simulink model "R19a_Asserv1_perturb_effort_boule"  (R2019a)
settings: Solver=ode15s  StartTime=0.0  StopTime=1  RelTol=1e-3  EnableMultiTasking=on
undefined symbols (not defined in the file): deg, kg, m, manette1_Défaut_sldprt, manette2_Défaut_sldprt, mm, N, rad, s, sigbuilder_block, STL, X, Y, Z
libraries: sm_lib x460, fl_lib x45, nesl_utility x23, simulink x3
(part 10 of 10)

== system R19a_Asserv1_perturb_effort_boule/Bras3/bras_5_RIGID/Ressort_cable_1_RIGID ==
  ReferenceFrame : sm_lib/Frames and Transforms/Reference Frame
  Solid : sm_lib/Body Elements/Solid  InertiaType=Custom  Mass=0.0011765814520035881  MassUnits=kg  CenterOfMass=[0.086849073647483815 -0.00090479521327996976 6.9508776157243597]  CenterOfMassUnits=mm  MomentsOfInertia=[0.034952381374405594 0.034338972761516762 0.0097063586011258158]  MomentsOfInertiaUnits=kg*mm^2  ProductsOfInertia=[0.00037229322226744533 1.6947615167207185e-06 2.0937803976811866e-06]  ProductsOfInertiaUnits=kg*mm^2  BasedOnType=Density  Density=1000  DensityUnits=kg/(m^3)  DoExposeReferenceFrame=on  SerializedFrames=<Frames/>  GraphicType=FromGeometry  MarkerShape=Sphere  MarkerSize=10  MarkerSizeUnits=m  GraphicVisPropType=SimpleVisualProperties  GraphicDiffuseColor=[0.6470588235294118 0.61960784313725492 0.58823529411764708]  GraphicSpecularColor=[0.5 0.5 0.5 1.0]  GraphicAmbientColor=[0.15 0.15 0.15 1.0]  GraphicEmissiveColor=[0.0 0.0 0.0 1.0]  GraphicShininess=75  GraphicOpacity=1  GeometryShape=FromFile  RectangleSize=[1 1]  RectangleSizeUnits=m  BrickDimensions=[1 1 1]  BrickDimensionUnits=m  CylinderRadius=1  CylinderRadiusUnits=m  CylinderLength=1  CylinderLengthUnits=m  SphereRadius=1  SphereRadiusUnits=m  EllipsoidRadii=[1 1 1]  EllipsoidRadiiUnits=m  ExtrusionCrossSection=[1 1; -1 1; -1 -1; 1 -1]  ExtrusionCrossSectionUnits=m  ExtrusionLength=1  ExtrusionLengthUnits=m  PolygonNumSides=3  PolygonOuterRadius=1  PolygonOuterRadiusUnits=m  ExtGeomFileType=STL  ExtGeomFileName=\STL\Ressort cable_Défaut_sldprt.STL  ExtGeomFileUnits=mm  RevolutionCrossSection=[1 1; 1 -1; 2 -1; 2 1]  RevolutionCrossSectionUnits=m  RevolutionExtent=Full  RevolutionAngle=180  RevolutionAngleUnits=deg
  F : PMIOPort  Side=Left
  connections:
  Solid/RConn1 -- ReferenceFrame/RConn1 -- F/RConn1

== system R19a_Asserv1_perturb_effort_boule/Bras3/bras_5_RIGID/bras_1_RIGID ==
  ReferenceFrame : sm_lib/Frames and Transforms/Reference Frame
  Solid : sm_lib/Body Elements/Solid  InertiaType=Custom  Mass=0.06566875822643542  MassUnits=kg  CenterOfMass=[23.925748169887701 -4.7774352723885904 0.0071346362933715022]  CenterOfMassUnits=mm  MomentsOfInertia=[75.153076467382206 23.577652078949701 94.231108050856861]  MomentsOfInertiaUnits=kg*mm^2  ProductsOfInertia=[0.01532312637695204 0.0017211125494294708 -5.8798668472039237]  ProductsOfInertiaUnits=kg*mm^2  BasedOnType=Density  Density=1000  DensityUnits=kg/(m^3)  DoExposeReferenceFrame=on  SerializedFrames=<Frames/>  GraphicType=FromGeometry  MarkerShape=Sphere  MarkerSize=10  MarkerSizeUnits=m  GraphicVisPropType=SimpleVisualProperties  GraphicDiffuseColor=[1.0 1.0 0.0]  GraphicSpecularColor=[0.5 0.5 0.5 1.0]  GraphicAmbientColor=[0.15 0.15 0.15 1.0]  GraphicEmissiveColor=[0.0 0.0 0.0 1.0]  GraphicShininess=75  GraphicOpacity=1  GeometryShape=FromFile  RectangleSize=[1 1]  RectangleSizeUnits=m  BrickDimensions=[1 1 1]  BrickDimensionUnits=m  CylinderRadius=1  CylinderRadiusUnits=m  CylinderLength=1  CylinderLengthUnits=m  SphereRadius=1  SphereRadiusUnits=m  EllipsoidRadii=[1 1 1]  EllipsoidRadiiUnits=m  ExtrusionCrossSection=[1 1; -1 1; -1 -1; 1 -1]  ExtrusionCrossSectionUnits=m  ExtrusionLength=1  ExtrusionLengthUnits=m  PolygonNumSides=3  PolygonOuterRadius=1  PolygonOuterRadiusUnits=m  ExtGeomFileType=STL  ExtGeomFileName=\STL\bras_Défaut_sldprt.STL  ExtGeomFileUnits=mm  RevolutionCrossSection=[1 1; 1 -1; 2 -1; 2 1]  RevolutionCrossSectionUnits=m  RevolutionExtent=Full  RevolutionAngle=180  RevolutionAngleUnits=deg
  F : PMIOPort  Side=Left
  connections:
  Solid/RConn1 -- ReferenceFrame/RConn1 -- F/RConn1

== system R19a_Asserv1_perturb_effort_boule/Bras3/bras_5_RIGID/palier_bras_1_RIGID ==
  ReferenceFrame : sm_lib/Frames and Transforms/Reference Frame
  Solid : sm_lib/Body Elements/Solid  InertiaType=Custom  Mass=0.00017920168094851793  MassUnits=kg  CenterOfMass=[-178.32667601154176 39.825618202078154 -20.980989744703667]  CenterOfMassUnits=mm  MomentsOfInertia=[0.0018602253674838991 0.0012789874237151958 0.0012789874237151961]  MomentsOfInertiaUnits=kg*mm^2  ProductsOfInertia=[0 0 0]  ProductsOfInertiaUnits=kg*mm^2  BasedOnType=Density  Density=1000  DensityUnits=kg/(m^3)  DoExposeReferenceFrame=on  SerializedFrames=<Frames/>  GraphicType=FromGeometry  MarkerShape=Sphere  MarkerSize=10  MarkerSizeUnits=m  GraphicVisPropType=SimpleVisualProperties  GraphicDiffuseColor=[1 1 1]  GraphicSpecularColor=[0.5 0.5 0.5 1.0]  GraphicAmbientColor=[0.15 0.15 0.15 1.0]  GraphicEmissiveColor=[0.0 0.0 0.0 1.0]  GraphicShininess=75  GraphicOpacity=1  GeometryShape=FromFile  RectangleSize=[1 1]  RectangleSizeUnits=m  BrickDimensions=[1 1 1]  BrickDimensionUnits=m  CylinderRadius=1  CylinderRadiusUnits=m  CylinderLength=1  CylinderLengthUnits=m  SphereRadius=1  SphereRadiusUnits=m  EllipsoidRadii=[1 1 1]  EllipsoidRadiiUnits=m  ExtrusionCrossSection=[1 1; -1 1; -1 -1; 1 -1]  ExtrusionCrossSectionUnits=m  ExtrusionLength=1  ExtrusionLengthUnits=m  PolygonNumSides=3  PolygonOuterRadius=1  PolygonOuterRadiusUnits=m  ExtGeomFileType=STL  ExtGeomFileName=\STL\palier bras_Défaut_sldprt.STL  ExtGeomFileUnits=mm  RevolutionCrossSection=[1 1; 1 -1; 2 -1; 2 1]  RevolutionCrossSectionUnits=m  RevolutionExtent=Full  RevolutionAngle=180  RevolutionAngleUnits=deg
  F : PMIOPort  Side=Left
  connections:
  Solid/RConn1 -- ReferenceFrame/RConn1 -- F/RConn1

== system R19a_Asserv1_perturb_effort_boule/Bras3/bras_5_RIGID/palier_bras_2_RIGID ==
  ReferenceFrame : sm_lib/Frames and Transforms/Reference Frame
  Solid : sm_lib/Body Elements/Solid  InertiaType=Custom  Mass=0.00017920168094851793  MassUnits=kg  CenterOfMass=[-178.32667601154176 39.825618202078154 -20.980989744703667]  CenterOfMassUnits=mm  MomentsOfInertia=[0.0018602253674838991 0.0012789874237151958 0.0012789874237151961]  MomentsOfInertiaUnits=kg*mm^2  ProductsOfInertia=[0 0 0]  ProductsOfInertiaUnits=kg*mm^2  BasedOnType=Density  Density=1000  DensityUnits=kg/(m^3)  DoExposeReferenceFrame=on  SerializedFrames=<Frames/>  GraphicType=FromGeometry  MarkerShape=Sphere  MarkerSize=10  MarkerSizeUnits=m  GraphicVisPropType=SimpleVisualProperties  GraphicDiffuseColor=[1 1 1]  GraphicSpecularColor=[0.5 0.5 0.5 1.0]  GraphicAmbientColor=[0.15 0.15 0.15 1.0]  GraphicEmissiveColor=[0.0 0.0 0.0 1.0]  GraphicShininess=75  GraphicOpacity=1  GeometryShape=FromFile  RectangleSize=[1 1]  RectangleSizeUnits=m  BrickDimensions=[1 1 1]  BrickDimensionUnits=m  CylinderRadius=1  CylinderRadiusUnits=m  CylinderLength=1  CylinderLengthUnits=m  SphereRadius=1  SphereRadiusUnits=m  EllipsoidRadii=[1 1 1]  EllipsoidRadiiUnits=m  ExtrusionCrossSection=[1 1; -1 1; -1 -1; 1 -1]  ExtrusionCrossSectionUnits=m  ExtrusionLength=1  ExtrusionLengthUnits=m  PolygonNumSides=3  PolygonOuterRadius=1  PolygonOuterRadiusUnits=m  ExtGeomFileType=STL  ExtGeomFileName=\STL\palier bras_Défaut_sldprt.STL  ExtGeomFileUnits=mm  RevolutionCrossSection=[1 1; 1 -1; 2 -1; 2 1]  RevolutionCrossSectionUnits=m  RevolutionExtent=Full  RevolutionAngle=180  RevolutionAngleUnits=deg
  F : PMIOPort  Side=Left
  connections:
  Solid/RConn1 -- ReferenceFrame/RConn1 -- F/RConn1

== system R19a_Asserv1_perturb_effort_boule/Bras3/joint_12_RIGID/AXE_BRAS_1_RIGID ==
  ReferenceFrame : sm_lib/Frames and Transforms/Reference Frame
  Solid : sm_lib/Body Elements/Solid  InertiaType=Custom  Mass=0.0015327306958088996  MassUnits=kg  CenterOfMass=[0 0 0]  CenterOfMassUnits=mm  MomentsOfInertia=[0.11359646260705632 0.11359646260705632 0.0017137152305883286]  MomentsOfInertiaUnits=kg*mm^2  ProductsOfInertia=[0 0 0]  ProductsOfInertiaUnits=kg*mm^2  BasedOnType=Density  Density=1000  DensityUnits=kg/(m^3)  DoExposeReferenceFrame=on  SerializedFrames=<Frames/>  GraphicType=FromGeometry  MarkerShape=Sphere  MarkerSize=10  MarkerSizeUnits=m  GraphicVisPropType=SimpleVisualProperties  GraphicDiffuseColor=[0.6470588235294118 0.61960784313725492 0.58823529411764708]  GraphicSpecularColor=[0.5 0.5 0.5 1.0]  GraphicAmbientColor=[0.15 0.15 0.15 1.0]  GraphicEmissiveColor=[0.0 0.0 0.0 1.0]  GraphicShininess=75  GraphicOpacity=1  GeometryShape=FromFile  RectangleSize=[1 1]  RectangleSizeUnits=m  BrickDimensions=[1 1 1]  BrickDimensionUnits=m  CylinderRadius=1  CylinderRadiusUnits=m  CylinderLength=1  CylinderLengthUnits=m  SphereRadius=1  SphereRadiusUnits=m  EllipsoidRadii=[1 1 1]  EllipsoidRadiiUnits=m  ExtrusionCrossSection=[1 1; -1 1; -1 -1; 1 -1]  ExtrusionCrossSectionUnits=m  ExtrusionLength=1  ExtrusionLengthUnits=m  PolygonNumSides=3  PolygonOuterRadius=1  PolygonOuterRadiusUnits=m  ExtGeomFileType=STL  ExtGeomFileName=\STL\AXE BRAS_Défaut_sldprt.STL  ExtGeomFileUnits=mm  RevolutionCrossSection=[1 1; 1 -1; 2 -1; 2 1]  RevolutionCrossSectionUnits=m  RevolutionExtent=Full  RevolutionAngle=180  RevolutionAngleUnits=deg
  F : PMIOPort  Side=Left
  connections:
  Solid/RConn1 -- ReferenceFrame/RConn1 -- F/RConn1

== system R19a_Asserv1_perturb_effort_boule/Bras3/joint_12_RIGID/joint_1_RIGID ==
  ReferenceFrame : sm_lib/Frames and Transforms/Reference Frame
  Solid : sm_lib/Body Elements/Solid  InertiaType=Custom  Mass=0.0062454336323428689  MassUnits=kg  CenterOfMass=[-4.7519597301086606e-06 14.873568128586268 0.2827021501004604]  CenterOfMassUnits=mm  MomentsOfInertia=[0.43544209184236687 0.81590742360241675 0.91424830357082487]  MomentsOfInertiaUnits=kg*mm^2  ProductsOfInertia=[0.0068320776316595647 -4.173068650825101e-06 -7.5142319098046527e-07]  ProductsOfInertiaUnits=kg*mm^2  BasedOnType=Density  Density=1000  DensityUnits=kg/(m^3)  DoExposeReferenceFrame=on  SerializedFrames=<Frames/>  GraphicType=FromGeometry  MarkerShape=Sphere  MarkerSize=10  MarkerSizeUnits=m  GraphicVisPropType=SimpleVisualProperties  GraphicDiffuseColor=[1 1 1]  GraphicSpecularColor=[0.5 0.5 0.5 1.0]  GraphicAmbientColor=[0.15 0.15 0.15 1.0]  GraphicEmissiveColor=[0.0 0.0 0.0 1.0]  GraphicShininess=75  GraphicOpacity=1  GeometryShape=FromFile  RectangleSize=[1 1]  RectangleSizeUnits=m  BrickDimensions=[1 1 1]  BrickDimensionUnits=m  CylinderRadius=1  CylinderRadiusUnits=m  CylinderLength=1  CylinderLengthUnits=m  SphereRadius=1  SphereRadiusUnits=m  EllipsoidRadii=[1 1 1]  EllipsoidRadiiUnits=m  ExtrusionCrossSection=[1 1; -1 1; -1 -1; 1 -1]  ExtrusionCrossSectionUnits=m  ExtrusionLength=1  ExtrusionLengthUnits=m  PolygonNumSides=3  PolygonOuterRadius=1  PolygonOuterRadiusUnits=m  ExtGeomFileType=STL  ExtGeomFileName=\STL\joint_Défaut_sldprt.STL  ExtGeomFileUnits=mm  RevolutionCrossSection=[1 1; 1 -1; 2 -1; 2 1]  RevolutionCrossSectionUnits=m  RevolutionExtent=Full  RevolutionAngle=180  RevolutionAngleUnits=deg
  F : PMIOPort  Side=Left
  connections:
  Solid/RConn1 -- ReferenceFrame/RConn1 -- F/RConn1

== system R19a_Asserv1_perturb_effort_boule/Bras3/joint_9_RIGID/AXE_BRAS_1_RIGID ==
  ReferenceFrame : sm_lib/Frames and Transforms/Reference Frame
  Solid : sm_lib/Body Elements/Solid  InertiaType=Custom  Mass=0.0015327306958088996  MassUnits=kg  CenterOfMass=[0 0 0]  CenterOfMassUnits=mm  MomentsOfInertia=[0.11359646260705632 0.11359646260705632 0.0017137152305883286]  MomentsOfInertiaUnits=kg*mm^2  ProductsOfInertia=[0 0 0]  ProductsOfInertiaUnits=kg*mm^2  BasedOnType=Density  Density=1000  DensityUnits=kg/(m^3)  DoExposeReferenceFrame=on  SerializedFrames=<Frames/>  GraphicType=FromGeometry  MarkerShape=Sphere  MarkerSize=10  MarkerSizeUnits=m  GraphicVisPropType=SimpleVisualProperties  GraphicDiffuseColor=[0.6470588235294118 0.61960784313725492 0.58823529411764708]  GraphicSpecularColor=[0.5 0.5 0.5 1.0]  GraphicAmbientColor=[0.15 0.15 0.15 1.0]  GraphicEmissiveColor=[0.0 0.0 0.0 1.0]  GraphicShininess=75  GraphicOpacity=1  GeometryShape=FromFile  RectangleSize=[1 1]  RectangleSizeUnits=m  BrickDimensions=[1 1 1]  BrickDimensionUnits=m  CylinderRadius=1  CylinderRadiusUnits=m  CylinderLength=1  CylinderLengthUnits=m  SphereRadius=1  SphereRadiusUnits=m  EllipsoidRadii=[1 1 1]  EllipsoidRadiiUnits=m  ExtrusionCrossSection=[1 1; -1 1; -1 -1; 1 -1]  ExtrusionCrossSectionUnits=m  ExtrusionLength=1  ExtrusionLengthUnits=m  PolygonNumSides=3  PolygonOuterRadius=1  PolygonOuterRadiusUnits=m  ExtGeomFileType=STL  ExtGeomFileName=\STL\AXE BRAS_Défaut_sldprt.STL  ExtGeomFileUnits=mm  RevolutionCrossSection=[1 1; 1 -1; 2 -1; 2 1]  RevolutionCrossSectionUnits=m  RevolutionExtent=Full  RevolutionAngle=180  RevolutionAngleUnits=deg
  F : PMIOPort  Side=Left
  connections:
  Solid/RConn1 -- ReferenceFrame/RConn1 -- F/RConn1

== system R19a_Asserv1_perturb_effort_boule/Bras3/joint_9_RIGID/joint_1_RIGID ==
  ReferenceFrame : sm_lib/Frames and Transforms/Reference Frame
  Solid : sm_lib/Body Elements/Solid  InertiaType=Custom  Mass=0.0062454336323428689  MassUnits=kg  CenterOfMass=[-4.7519597301086606e-06 14.873568128586268 0.2827021501004604]  CenterOfMassUnits=mm  MomentsOfInertia=[0.43544209184236687 0.81590742360241675 0.91424830357082487]  MomentsOfInertiaUnits=kg*mm^2  ProductsOfInertia=[0.0068320776316595647 -4.173068650825101e-06 -7.5142319098046527e-07]  ProductsOfInertiaUnits=kg*mm^2  BasedOnType=Density  Density=1000  DensityUnits=kg/(m^3)  DoExposeReferenceFrame=on  SerializedFrames=<Frames/>  GraphicType=FromGeometry  MarkerShape=Sphere  MarkerSize=10  MarkerSizeUnits=m  GraphicVisPropType=SimpleVisualProperties  GraphicDiffuseColor=[1 1 1]  GraphicSpecularColor=[0.5 0.5 0.5 1.0]  GraphicAmbientColor=[0.15 0.15 0.15 1.0]  GraphicEmissiveColor=[0.0 0.0 0.0 1.0]  GraphicShininess=75  GraphicOpacity=1  GeometryShape=FromFile  RectangleSize=[1 1]  RectangleSizeUnits=m  BrickDimensions=[1 1 1]  BrickDimensionUnits=m  CylinderRadius=1  CylinderRadiusUnits=m  CylinderLength=1  CylinderLengthUnits=m  SphereRadius=1  SphereRadiusUnits=m  EllipsoidRadii=[1 1 1]  EllipsoidRadiiUnits=m  ExtrusionCrossSection=[1 1; -1 1; -1 -1; 1 -1]  ExtrusionCrossSectionUnits=m  ExtrusionLength=1  ExtrusionLengthUnits=m  PolygonNumSides=3  PolygonOuterRadius=1  PolygonOuterRadiusUnits=m  ExtGeomFileType=STL  ExtGeomFileName=\STL\joint_Défaut_sldprt.STL  ExtGeomFileUnits=mm  RevolutionCrossSection=[1 1; 1 -1; 2 -1; 2 1]  RevolutionCrossSectionUnits=m  RevolutionExtent=Full  RevolutionAngle=180  RevolutionAngleUnits=deg
  F : PMIOPort  Side=Left
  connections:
  Solid/RConn1 -- ReferenceFrame/RConn1 -- F/RConn1

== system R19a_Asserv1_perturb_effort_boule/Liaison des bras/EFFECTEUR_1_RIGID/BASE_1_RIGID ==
  ReferenceFrame : sm_lib/Frames and Transforms/Reference Frame
  Solid : sm_lib/Body Elements/Solid  InertiaType=Custom  Mass=0.028238598075005058  MassUnits=kg  CenterOfMass=[-0.50940754911928388 -1.6318221689243708 -4.5607511741024656]  CenterOfMassUnits=mm  MomentsOfInertia=[8.5842414198569479 7.5819347196129669 14.129620619032369]  MomentsOfInertiaUnits=kg*mm^2  ProductsOfInertia=[-0.29549774773685261 -0.082418003511546406 -0.14811223553088118]  ProductsOfInertiaUnits=kg*mm^2  BasedOnType=Density  Density=1000  DensityUnits=kg/(m^3)  DoExposeReferenceFrame=on  SerializedFrames=<Frames/>  GraphicType=FromGeometry  MarkerShape=Sphere  MarkerSize=10  MarkerSizeUnits=m  GraphicVisPropType=SimpleVisualProperties  GraphicDiffuseColor=[1.0 1.0 1.0]  GraphicSpecularColor=[0.5 0.5 0.5 1.0]  GraphicAmbientColor=[0.15 0.15 0.15 1.0]  GraphicEmissiveColor=[0.0 0.0 0.0 1.0]  GraphicShininess=75  GraphicOpacity=1  GeometryShape=FromFile  RectangleSize=[1 1]  RectangleSizeUnits=m  BrickDimensions=[1 1 1]  BrickDimensionUnits=m  CylinderRadius=1  CylinderRadiusUnits=m  CylinderLength=1  CylinderLengthUnits=m  SphereRadius=1  SphereRadiusUnits=m  EllipsoidRadii=[1 1 1]  EllipsoidRadiiUnits=m  ExtrusionCrossSection=[1 1; -1 1; -1 -1; 1 -1]  ExtrusionCrossSectionUnits=m  ExtrusionLength=1  ExtrusionLengthUnits=m  PolygonNumSides=3  PolygonOuterRadius=1  PolygonOuterRadiusUnits=m  ExtGeomFileType=STL  ExtGeomFileName=\STL\BASE_Défaut_sldprt.STL  ExtGeomFileUnits=mm  RevolutionCrossSection=[1 1; 1 -1; 2 -1; 2 1]  RevolutionCrossSectionUnits=m  RevolutionExtent=Full  RevolutionAngle=180  RevolutionAngleUnits=deg
  F : PMIOPort  Side=Left
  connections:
  Solid/RConn1 -- ReferenceFrame/RConn1 -- F/RConn1

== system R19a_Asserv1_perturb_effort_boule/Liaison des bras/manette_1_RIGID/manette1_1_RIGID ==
  ReferenceFrame : sm_lib/Frames and Transforms/Reference Frame
  Solid : sm_lib/Body Elements/Solid  InertiaType=Custom  Mass=0.021495200046783486  MassUnits=kg  CenterOfMass=[-1.4897475291331288 1.1324325333899619 3.6124835128376875]  CenterOfMassUnits=mm  MomentsOfInertia=[5.4184345928892519 5.4614392106741905 10.048915162120133]  MomentsOfInertiaUnits=kg*mm^2  ProductsOfInertia=[-0.010452851512005331 -0.0018797921399214363 0.024517118393881449]  ProductsOfInertiaUnits=kg*mm^2  BasedOnType=Density  Density=1000  DensityUnits=kg/(m^3)  DoExposeReferenceFrame=on  SerializedFrames=<Frames/>  GraphicType=FromGeometry  MarkerShape=Sphere  MarkerSize=10  MarkerSizeUnits=m  GraphicVisPropType=SimpleVisualProperties  GraphicDiffuseColor=[0.8 0.8 0.8]  GraphicSpecularColor=[0.5 0.5 0.5 1.0]  GraphicAmbientColor=[0.15 0.15 0.15 1.0]  GraphicEmissiveColor=[0.0 0.0 0.0 1.0]  GraphicShininess=75  GraphicOpacity=1  GeometryShape=FromFile  RectangleSize=[1 1]  RectangleSizeUnits=m  BrickDimensions=[1 1 1]  BrickDimensionUnits=m  CylinderRadius=1  CylinderRadiusUnits=m  CylinderLength=1  CylinderLengthUnits=m  SphereRadius=1  SphereRadiusUnits=m  EllipsoidRadii=[1 1 1]  EllipsoidRadiiUnits=m  ExtrusionCrossSection=[1 1; -1 1; -1 -1; 1 -1]  ExtrusionCrossSectionUnits=m  ExtrusionLength=1  ExtrusionLengthUnits=m  PolygonNumSides=3  PolygonOuterRadius=1  PolygonOuterRadiusUnits=m  ExtGeomFileType=STL  ExtGeomFileName=\STL\manette1_Défaut_sldprt.STL  ExtGeomFileUnits=mm  RevolutionCrossSection=[1 1; 1 -1; 2 -1; 2 1]  RevolutionCrossSectionUnits=m  RevolutionExtent=Full  RevolutionAngle=180  RevolutionAngleUnits=deg
  F : PMIOPort  Side=Left
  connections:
  Solid/RConn1 -- ReferenceFrame/RConn1 -- F/RConn1

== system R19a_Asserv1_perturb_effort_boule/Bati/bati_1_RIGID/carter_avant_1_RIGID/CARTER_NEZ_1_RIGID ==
  ReferenceFrame : sm_lib/Frames and Transforms/Reference Frame
  Solid : sm_lib/Body Elements/Solid  InertiaType=Custom  Mass=0.023684568109850399  MassUnits=kg  CenterOfMass=[17.102684932647009 114.0476537917955 1.3404873933864438]  CenterOfMassUnits=mm  MomentsOfInertia=[16.43130676036915 32.571595129912247 16.431105891514132]  MomentsOfInertiaUnits=kg*mm^2  ProductsOfInertia=[-3.788014627850142e-05 -4.8452777139477129e-05 -5.4026210558728518e-06]  ProductsOfInertiaUnits=kg*mm^2  BasedOnType=Density  Density=1000  DensityUnits=kg/(m^3)  DoExposeReferenceFrame=on  SerializedFrames=<Frames/>  GraphicType=FromGeometry  MarkerShape=Sphere  MarkerSize=10  MarkerSizeUnits=m  GraphicVisPropType=SimpleVisualProperties  GraphicDiffuseColor=[0.75294117647058822 0.75294117647058822 0.75294117647058822]  GraphicSpecularColor=[0.5 0.5 0.5 1.0]  GraphicAmbientColor=[0.15 0.15 0.15 1.0]  GraphicEmissiveColor=[0.0 0.0 0.0 1.0]  GraphicShininess=75  GraphicOpacity=1  GeometryShape=FromFile  RectangleSize=[1 1]  RectangleSizeUnits=m  BrickDimensions=[1 1 1]  BrickDimensionUnits=m  CylinderRadius=1  CylinderRadiusUnits=m  CylinderLength=1  CylinderLengthUnits=m  SphereRadius=1  SphereRadiusUnits=m  EllipsoidRadii=[1 1 1]  EllipsoidRadiiUnits=m  ExtrusionCrossSection=[1 1; -1 1; -1 -1; 1 -1]  ExtrusionCrossSectionUnits=m  ExtrusionLength=1  ExtrusionLengthUnits=m  PolygonNumSides=3  PolygonOuterRadius=1  PolygonOuterRadiusUnits=m  ExtGeomFileType=STL  ExtGeomFileName=\STL\CARTER NEZ_Défaut_sldprt.STL  ExtGeomFileUnits=mm  RevolutionCrossSection=[1 1; 1 -1; 2 -1; 2 1]  RevolutionCrossSectionUnits=m  RevolutionExtent=Full  RevolutionAngle=180  RevolutionAngleUnits=deg
  F : PMIOPort  Side=Left
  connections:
  Solid/RConn1 -- ReferenceFrame/RConn1 -- F/RConn1

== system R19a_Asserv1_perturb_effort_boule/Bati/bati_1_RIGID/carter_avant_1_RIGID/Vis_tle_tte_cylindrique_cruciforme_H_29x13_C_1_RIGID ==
  ReferenceFrame : sm_lib/Frames and Transforms/Reference Frame
  Solid : sm_lib/Body Elements/Solid  InertiaType=Custom  Mass=8.3821869835456372e-05  MassUnits=kg  CenterOfMass=[4.9478681581074904 0.00064910481891303923 -0.0013634218224953438]  CenterOfMassUnits=mm  MomentsOfInertia=[0.00016543197172893975 0.0014334630955093895 0.0014333390308476422]  MomentsOfInertiaUnits=kg*mm^2  ProductsOfInertia=[-5.4062904633677868e-09 -1.3111174919527308e-07 6.0713893531177014e-07]  ProductsOfInertiaUnits=kg*mm^2  BasedOnType=Density  Density=1000  DensityUnits=kg/(m^3)  DoExposeReferenceFrame=on  SerializedFrames=<Frames/>  GraphicType=FromGeometry  MarkerShape=Sphere  MarkerSize=10  MarkerSizeUnits=m  GraphicVisPropType=SimpleVisualProperties  GraphicDiffuseColor=[0.75294117647058822 0.75294117647058822 0.75294117647058822]  GraphicSpecularColor=[0.5 0.5 0.5 1.0]  GraphicAmbientColor=[0.15 0.15 0.15 1.0]  GraphicEmissiveColor=[0.0 0.0 0.0 1.0]  GraphicShininess=75  GraphicOpacity=1  GeometryShape=FromFile  RectangleSize=[1 1]  RectangleSizeUnits=m  BrickDimensions=[1 1 1]  BrickDimensionUnits=m  CylinderRadius=1  CylinderRadiusUnits=m  CylinderLength=1  CylinderLengthUnits=m  SphereRadius=1  SphereRadiusUnits=m  EllipsoidRadii=[1 1 1]  EllipsoidRadiiUnits=m  ExtrusionCrossSection=[1 1; -1 1; -1 -1; 1 -1]  ExtrusionCrossSectionUnits=m  ExtrusionLength=1  ExtrusionLengthUnits=m  PolygonNumSides=3  PolygonOuterRadius=1  PolygonOuterRadiusUnits=m  ExtGeomFileType=STL  ExtGeomFileName=\STL\Vis à tôle tête cylindrique cruciforme H 2-9x13 - C_Réaliste_sldprt.STL  ExtGeomFileUnits=mm  RevolutionCrossSection=[1 1; 1 -1; 2 -1; 2 1]  RevolutionCrossSectionUnits=m  RevolutionExtent=Full  RevolutionAngle=180  RevolutionAngleUnits=deg
  F : PMIOPort  Side=Left
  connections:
  Solid/RConn1 -- ReferenceFrame/RConn1 -- F/RConn1

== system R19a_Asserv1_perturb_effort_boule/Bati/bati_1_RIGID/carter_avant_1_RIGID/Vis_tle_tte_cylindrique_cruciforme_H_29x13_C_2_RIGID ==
  ReferenceFrame : sm_lib/Frames and Transforms/Reference Frame
  Solid : sm_lib/Body Elements/Solid  InertiaType=Custom  Mass=8.3821869835456372e-05  MassUnits=kg  CenterOfMass=[4.9478681581074904 0.00064910481891303923 -0.0013634218224953438]  CenterOfMassUnits=mm  MomentsOfInertia=[0.00016543197172893975 0.0014334630955093895 0.0014333390308476422]  MomentsOfInertiaUnits=kg*mm^2  ProductsOfInertia=[-5.4062904633677868e-09 -1.3111174919527308e-07 6.0713893531177014e-07]  ProductsOfInertiaUnits=kg*mm^2  BasedOnType=Density  Density=1000  DensityUnits=kg/(m^3)  DoExposeReferenceFrame=on  SerializedFrames=<Frames/>  GraphicType=FromGeometry  MarkerShape=Sphere  MarkerSize=10  MarkerSizeUnits=m  GraphicVisPropType=SimpleVisualProperties  GraphicDiffuseColor=[0.75294117647058822 0.75294117647058822 0.75294117647058822]  GraphicSpecularColor=[0.5 0.5 0.5 1.0]  GraphicAmbientColor=[0.15 0.15 0.15 1.0]  GraphicEmissiveColor=[0.0 0.0 0.0 1.0]  GraphicShininess=75  GraphicOpacity=1  GeometryShape=FromFile  RectangleSize=[1 1]  RectangleSizeUnits=m  BrickDimensions=[1 1 1]  BrickDimensionUnits=m  CylinderRadius=1  CylinderRadiusUnits=m  CylinderLength=1  CylinderLengthUnits=m  SphereRadius=1  SphereRadiusUnits=m  EllipsoidRadii=[1 1 1]  EllipsoidRadiiUnits=m  ExtrusionCrossSection=[1 1; -1 1; -1 -1; 1 -1]  ExtrusionCrossSectionUnits=m  ExtrusionLength=1  ExtrusionLengthUnits=m  PolygonNumSides=3  PolygonOuterRadius=1  PolygonOuterRadiusUnits=m  ExtGeomFileType=STL  ExtGeomFileName=\STL\Vis à tôle tête cylindrique cruciforme H 2-9x13 - C_Réaliste_sldprt.STL  ExtGeomFileUnits=mm  RevolutionCrossSection=[1 1; 1 -1; 2 -1; 2 1]  RevolutionCrossSectionUnits=m  RevolutionExtent=Full  RevolutionAngle=180  RevolutionAngleUnits=deg
  F : PMIOPort  Side=Left
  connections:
  Solid/RConn1 -- ReferenceFrame/RConn1 -- F/RConn1

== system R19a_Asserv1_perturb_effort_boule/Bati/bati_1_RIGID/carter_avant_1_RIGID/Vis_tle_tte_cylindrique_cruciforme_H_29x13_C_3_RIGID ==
  ReferenceFrame : sm_lib/Frames and Transforms/Reference Frame
  Solid : sm_lib/Body Elements/Solid  InertiaType=Custom  Mass=8.3821869835456372e-05  MassUnits=kg  CenterOfMass=[4.9478681581074904 0.00064910481891303923 -0.0013634218224953438]  CenterOfMassUnits=mm  MomentsOfInertia=[0.00016543197172893975 0.0014334630955093895 0.0014333390308476422]  MomentsOfInertiaUnits=kg*mm^2  ProductsOfInertia=[-5.4062904633677868e-09 -1.3111174919527308e-07 6.0713893531177014e-07]  ProductsOfInertiaUnits=kg*mm^2  BasedOnType=Density  Density=1000  DensityUnits=kg/(m^3)  DoExposeReferenceFrame=on  SerializedFrames=<Frames/>  GraphicType=FromGeometry  MarkerShape=Sphere  MarkerSize=10  MarkerSizeUnits=m  GraphicVisPropType=SimpleVisualProperties  GraphicDiffuseColor=[0.75294117647058822 0.75294117647058822 0.75294117647058822]  GraphicSpecularColor=[0.5 0.5 0.5 1.0]  GraphicAmbientColor=[0.15 0.15 0.15 1.0]  GraphicEmissiveColor=[0.0 0.0 0.0 1.0]  GraphicShininess=75  GraphicOpacity=1  GeometryShape=FromFile  RectangleSize=[1 1]  RectangleSizeUnits=m  BrickDimensions=[1 1 1]  BrickDimensionUnits=m  CylinderRadius=1  CylinderRadiusUnits=m  CylinderLength=1  CylinderLengthUnits=m  SphereRadius=1  SphereRadiusUnits=m  EllipsoidRadii=[1 1 1]  EllipsoidRadiiUnits=m  ExtrusionCrossSection=[1 1; -1 1; -1 -1; 1 -1]  ExtrusionCrossSectionUnits=m  ExtrusionLength=1  ExtrusionLengthUnits=m  PolygonNumSides=3  PolygonOuterRadius=1  PolygonOuterRadiusUnits=m  ExtGeomFileType=STL  ExtGeomFileName=\STL\Vis à tôle tête cylindrique cruciforme H 2-9x13 - C_Réaliste_sldprt.STL  ExtGeomFileUnits=mm  RevolutionCrossSection=[1 1; 1 -1; 2 -1; 2 1]  RevolutionCrossSectionUnits=m  RevolutionExtent=Full  RevolutionAngle=180  RevolutionAngleUnits=deg
  F : PMIOPort  Side=Left
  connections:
  Solid/RConn1 -- ReferenceFrame/RConn1 -- F/RConn1

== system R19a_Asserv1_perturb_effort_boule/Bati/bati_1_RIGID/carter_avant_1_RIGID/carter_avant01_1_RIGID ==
  ReferenceFrame : sm_lib/Frames and Transforms/Reference Frame
  Solid : sm_lib/Body Elements/Solid  InertiaType=Custom  Mass=0.037834193553807655  MassUnits=kg  CenterOfMass=[-1.2122189045492688 175.43270841498617 61.584507438849911]  CenterOfMassUnits=mm  MomentsOfInertia=[56.040868119625912 128.12274252763086 98.880664351206846]  MomentsOfInertiaUnits=kg*mm^2  ProductsOfInertia=[17.771132404811137 -0.72051019684540141 0.93869411089982313]  ProductsOfInertiaUnits=kg*mm^2  BasedOnType=Density  Density=1000  DensityUnits=kg/(m^3)  DoExposeReferenceFrame=on  SerializedFrames=<Frames/>  GraphicType=FromGeometry  MarkerShape=Sphere  MarkerSize=10  MarkerSizeUnits=m  GraphicVisPropType=SimpleVisualProperties  GraphicDiffuseColor=[1.0 1.0 1.0]  GraphicSpecularColor=[0.5 0.5 0.5 1.0]  GraphicAmbientColor=[0.15 0.15 0.15 1.0]  GraphicEmissiveColor=[0.0 0.0 0.0 1.0]  GraphicShininess=75  GraphicOpacity=0  GeometryShape=FromFile  RectangleSize=[1 1]  RectangleSizeUnits=m  BrickDimensions=[1 1 1]  BrickDimensionUnits=m  CylinderRadius=1  CylinderRadiusUnits=m  CylinderLength=1  CylinderLengthUnits=m  SphereRadius=1  SphereRadiusUnits=m  EllipsoidRadii=[1 1 1]  EllipsoidRadiiUnits=m  ExtrusionCrossSection=[1 1; -1 1; -1 -1; 1 -1]  ExtrusionCrossSectionUnits=m  ExtrusionLength=1  ExtrusionLengthUnits=m  PolygonNumSides=3  PolygonOuterRadius=1  PolygonOuterRadiusUnits=m  ExtGeomFileType=STL  ExtGeomFileName=\STL\carter avant01_Défaut_sldprt.STL  ExtGeomFileUnits=mm  RevolutionCrossSection=[1 1; 1 -1; 2 -1; 2 1]  RevolutionCrossSectionUnits=m  RevolutionExtent=Full  RevolutionAngle=180  RevolutionAngleUnits=deg
  F : PMIOPort  Side=Left
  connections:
  Solid/RConn1 -- ReferenceFrame/RConn1 -- F/RConn1

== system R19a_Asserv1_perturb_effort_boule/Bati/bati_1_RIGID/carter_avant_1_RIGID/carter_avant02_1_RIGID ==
  ReferenceFrame : sm_lib/Frames and Transforms/Reference Frame
  Solid : sm_lib/Body Elements/Solid  InertiaType=Custom  Mass=0.04003612730019273  MassUnits=kg  CenterOfMass=[-5.5302874316411099 176.12322006317407 58.915594608725293]  CenterOfMassUnits=mm  MomentsOfInertia=[61.433722156029233 146.06754836858084 112.39719793476846]  MomentsOfInertiaUnits=kg*mm^2  ProductsOfInertia=[19.11954141989958 -8.6708453597958446 2.8769308330981094]  ProductsOfInertiaUnits=kg*mm^2  BasedOnType=Density  Density=1000  DensityUnits=kg/(m^3)  DoExposeReferenceFrame=on  SerializedFrames=<Frames/>  GraphicType=FromGeometry  MarkerShape=Sphere  MarkerSize=10  MarkerSizeUnits=m  GraphicVisPropType=SimpleVisualProperties  GraphicDiffuseColor=[1.0 1.0 1.0]  GraphicSpecularColor=[0.5 0.5 0.5 1.0]  GraphicAmbientColor=[0.15 0.15 0.15 1.0]  GraphicEmissiveColor=[0.0 0.0 0.0 1.0]  GraphicShininess=75  GraphicOpacity=1  GeometryShape=FromFile  RectangleSize=[1 1]  RectangleSizeUnits=m  BrickDimensions=[1 1 1]  BrickDimensionUnits=m  CylinderRadius=1  CylinderRadiusUnits=m  CylinderLength=1  CylinderLengthUnits=m  SphereRadius=1  SphereRadiusUnits=m  EllipsoidRadii=[1 1 1]  EllipsoidRadiiUnits=m  ExtrusionCrossSection=[1 1; -1 1; -1 -1; 1 -1]  ExtrusionCrossSectionUnits=m  ExtrusionLength=1  ExtrusionLengthUnits=m  PolygonNumSides=3  PolygonOuterRadius=1  PolygonOuterRadiusUnits=m  ExtGeomFileType=STL  ExtGeomFileName=\STL\carter avant02_Défaut_sldprt.STL  ExtGeomFileUnits=mm  RevolutionCrossSection=[1 1; 1 -1; 2 -1; 2 1]  RevolutionCrossSectionUnits=m  RevolutionExtent=Full  RevolutionAngle=180  RevolutionAngleUnits=deg
  F : PMIOPort  Side=Left
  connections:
  Solid/RConn1 -- ReferenceFrame/RConn1 -- F/RConn1

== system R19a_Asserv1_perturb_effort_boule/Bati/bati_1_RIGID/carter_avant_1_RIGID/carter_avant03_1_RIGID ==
  ReferenceFrame : sm_lib/Frames and Transforms/Reference Frame
  Solid : sm_lib/Body Elements/Solid  InertiaType=Custom  Mass=0.040033100851173897  MassUnits=kg  CenterOfMass=[3.2488267644133511 176.1208864671479 58.924212973359204]  CenterOfMassUnits=mm  MomentsOfInertia=[61.470691722682709 146.87719070674399 113.21967982116205]  MomentsOfInertiaUnits=kg*mm^2  ProductsOfInertia=[19.138525158618911 7.4477910669264711 -1.062715139795626]  ProductsOfInertiaUnits=kg*mm^2  BasedOnType=Density  Density=1000  DensityUnits=kg/(m^3)  DoExposeReferenceFrame=on  SerializedFrames=<Frames/>  GraphicType=FromGeometry  MarkerShape=Sphere  MarkerSize=10  MarkerSizeUnits=m  GraphicVisPropType=SimpleVisualProperties  GraphicDiffuseColor=[1.0 1.0 1.0]  GraphicSpecularColor=[0.5 0.5 0.5 1.0]  GraphicAmbientColor=[0.15 0.15 0.15 1.0]  GraphicEmissiveColor=[0.0 0.0 0.0 1.0]  GraphicShininess=75  GraphicOpacity=1  GeometryShape=FromFile  RectangleSize=[1 1]  RectangleSizeUnits=m  BrickDimensions=[1 1 1]  BrickDimensionUnits=m  CylinderRadius=1  CylinderRadiusUnits=m  CylinderLength=1  CylinderLengthUnits=m  SphereRadius=1  SphereRadiusUnits=m  EllipsoidRadii=[1 1 1]  EllipsoidRadiiUnits=m  ExtrusionCrossSection=[1 1; -1 1; -1 -1; 1 -1]  ExtrusionCrossSectionUnits=m  ExtrusionLength=1  ExtrusionLengthUnits=m  PolygonNumSides=3  PolygonOuterRadius=1  PolygonOuterRadiusUnits=m  ExtGeomFileType=STL  ExtGeomFileName=\STL\carter avant03_Défaut_sldprt.STL  ExtGeomFileUnits=mm  RevolutionCrossSection=[1 1; 1 -1; 2 -1; 2 1]  RevolutionCrossSectionUnits=m  RevolutionExtent=Full  RevolutionAngle=180  RevolutionAngleUnits=deg
  F : PMIOPort  Side=Left
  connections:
  Solid/RConn1 -- ReferenceFrame/RConn1 -- F/RConn1

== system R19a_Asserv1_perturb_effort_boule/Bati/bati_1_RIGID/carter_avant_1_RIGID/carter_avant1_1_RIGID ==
  ReferenceFrame : sm_lib/Frames and Transforms/Reference Frame
  Solid : sm_lib/Body Elements/Solid  InertiaType=Custom  Mass=0.0068977261305129805  MassUnits=kg  CenterOfMass=[0.013428833188053345 115.01841988578165 104.87566191405597]  CenterOfMassUnits=mm  MomentsOfInertia=[2.0334532747861105 2.0241587370426406 3.5278352594861393]  MomentsOfInertiaUnits=kg*mm^2  ProductsOfInertia=[-0.0020444395438733434 -2.1966864026409714e-05 -0.00053475799446389791]  ProductsOfInertiaUnits=kg*mm^2  BasedOnType=Density  Density=1000  DensityUnits=kg/(m^3)  DoExposeReferenceFrame=on  SerializedFrames=<Frames/>  GraphicType=FromGeometry  MarkerShape=Sphere  MarkerSize=10  MarkerSizeUnits=m  GraphicVisPropType=SimpleVisualProperties  GraphicDiffuseColor=[0.792156862745098 0.81960784313725488 0.93333333333333335]  GraphicSpecularColor=[0.5 0.5 0.5 1.0]  GraphicAmbientColor=[0.15 0.15 0.15 1.0]  GraphicEmissiveColor=[0.0 0.0 0.0 1.0]  GraphicShininess=75  GraphicOpacity=1  GeometryShape=FromFile  RectangleSize=[1 1]  RectangleSizeUnits=m  BrickDimensions=[1 1 1]  BrickDimensionUnits=m  CylinderRadius=1  CylinderRadiusUnits=m  CylinderLength=1  CylinderLengthUnits=m  SphereRadius=1  SphereRadiusUnits=m  EllipsoidRadii=[1 1 1]  EllipsoidRadiiUnits=m  ExtrusionCrossSection=[1 1; -1 1; -1 -1; 1 -1]  ExtrusionCrossSectionUnits=m  ExtrusionLength=1  ExtrusionLengthUnits=m  PolygonNumSides=3  PolygonOuterRadius=1  PolygonOuterRadiusUnits=m  ExtGeomFileType=STL  ExtGeomFileName=\STL\carter avant1_Défaut_sldprt.STL  ExtGeomFileUnits=mm  RevolutionCrossSection=[1 1; 1 -1; 2 -1; 2 1]  RevolutionCrossSectionUnits=m  RevolutionExtent=Full  RevolutionAngle=180  RevolutionAngleUnits=deg
  F : PMIOPort  Side=Left
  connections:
  Solid/RConn1 -- ReferenceFrame/RConn1 -- F/RConn1

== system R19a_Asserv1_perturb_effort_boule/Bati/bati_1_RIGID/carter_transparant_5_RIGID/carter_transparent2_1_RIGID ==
  ReferenceFrame : sm_lib/Frames and Transforms/Reference Frame
  Solid : sm_lib/Body Elements/Solid  InertiaType=Custom  Mass=0.09082975360372901  MassUnits=kg  CenterOfMass=[2.3301793536057773 71.397337965148168 56.68444733144738]  CenterOfMassUnits=mm  MomentsOfInertia=[150.08149768370154 164.27950343498205 187.86724715852677]  MomentsOfInertiaUnits=kg*mm^2  ProductsOfInertia=[-19.998213794105411 -3.3083924529632989 0.84436764044313561]  ProductsOfInertiaUnits=kg*mm^2  BasedOnType=Density  Density=1000  DensityUnits=kg/(m^3)  DoExposeReferenceFrame=on  SerializedFrames=<Frames/>  GraphicType=FromGeometry  MarkerShape=Sphere  MarkerSize=10  MarkerSizeUnits=m  GraphicVisPropType=SimpleVisualProperties  GraphicDiffuseColor=[0.792156862745098 0.81960784313725488 0.93333333333333335]  GraphicSpecularColor=[0.5 0.5 0.5 1.0]  GraphicAmbientColor=[0.15 0.15 0.15 1.0]  GraphicEmissiveColor=[0.0 0.0 0.0 1.0]  GraphicShininess=75  GraphicOpacity=1  GeometryShape=FromFile  RectangleSize=[1 1]  RectangleSizeUnits=m  BrickDimensions=[1 1 1]  BrickDimensionUnits=m  CylinderRadius=1  CylinderRadiusUnits=m  CylinderLength=1  CylinderLengthUnits=m  SphereRadius=1  SphereRadiusUnits=m  EllipsoidRadii=[1 1 1]  EllipsoidRadiiUnits=m  ExtrusionCrossSection=[1 1; -1 1; -1 -1; 1 -1]  ExtrusionCrossSectionUnits=m  ExtrusionLength=1  ExtrusionLengthUnits=m  PolygonNumSides=3  PolygonOuterRadius=1  PolygonOuterRadiusUnits=m  ExtGeomFileType=STL  ExtGeomFileName=\STL\carter transparent2_Défaut_sldprt.STL  ExtGeomFileUnits=mm  RevolutionCrossSection=[1 1; 1 -1; 2 -1; 2 1]  RevolutionCrossSectionUnits=m  RevolutionExtent=Full  RevolutionAngle=180  RevolutionAngleUnits=deg
  F : PMIOPort  Side=Left
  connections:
  Solid/RConn1 -- ReferenceFrame/RConn1 -- F/RConn1

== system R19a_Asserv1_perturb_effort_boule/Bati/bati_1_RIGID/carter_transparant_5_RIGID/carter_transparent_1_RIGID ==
  ReferenceFrame : sm_lib/Frames and Transforms/Reference Frame
  Solid : sm_lib/Body Elements/Solid  InertiaType=Custom  Mass=0.056273911834023478  MassUnits=kg  CenterOfMass=[12.60882798450937 60.199925046373778 61.212214588211637]  CenterOfMassUnits=mm  MomentsOfInertia=[58.20868427615801 95.569253812513907 86.337959151344037]  MomentsOfInertiaUnits=kg*mm^2  ProductsOfInertia=[-17.408508514500589 1.3730953848150378 -5.3261234176687369]  ProductsOfInertiaUnits=kg*mm^2  BasedOnType=Density  Density=1000  DensityUnits=kg/(m^3)  DoExposeReferenceFrame=on  SerializedFrames=<Frames/>  GraphicType=FromGeometry  MarkerShape=Sphere  MarkerSize=10  MarkerSizeUnits=m  GraphicVisPropType=SimpleVisualProperties  GraphicDiffuseColor=[0.792156862745098 0.81960784313725488 0.93333333333333335]  GraphicSpecularColor=[0.5 0.5 0.5 1.0]  GraphicAmbientColor=[0.15 0.15 0.15 1.0]  GraphicEmissiveColor=[0.0 0.0 0.0 1.0]  GraphicShininess=75  GraphicOpacity=1  GeometryShape=FromFile  RectangleSize=[1 1]  RectangleSizeUnits=m  BrickDimensions=[1 1 1]  BrickDimensionUnits=m  CylinderRadius=1  CylinderRadiusUnits=m  CylinderLength=1  CylinderLengthUnits=m  SphereRadius=1  SphereRadiusUnits=m  EllipsoidRadii=[1 1 1]  EllipsoidRadiiUnits=m  ExtrusionCrossSection=[1 1; -1 1; -1 -1; 1 -1]  ExtrusionCrossSectionUnits=m  ExtrusionLength=1  ExtrusionLengthUnits=m  PolygonNumSides=3  PolygonOuterRadius=1  PolygonOuterRadiusUnits=m  ExtGeomFileType=STL  ExtGeomFileName=\STL\carter transparent_Défaut_sldprt.STL  ExtGeomFileUnits=mm  RevolutionCrossSection=[1 1; 1 -1; 2 -1; 2 1]  RevolutionCrossSectionUnits=m  RevolutionExtent=Full  RevolutionAngle=180  RevolutionAngleUnits=deg
  F : PMIOPort  Side=Left
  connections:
  Solid/RConn1 -- ReferenceFrame/RConn1 -- F/RConn1

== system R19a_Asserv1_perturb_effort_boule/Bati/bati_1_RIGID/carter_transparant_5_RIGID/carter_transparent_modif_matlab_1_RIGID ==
  ReferenceFrame : sm_lib/Frames and Transforms/Reference Frame
  Solid : sm_lib/Body Elements/Solid  InertiaType=Custom  Mass=0.044889069172440496  MassUnits=kg  CenterOfMass=[-16.380945858412954 64.543634175323007 61.916354268852707]  CenterOfMassUnits=mm  MomentsOfInertia=[48.669303101169348 65.98246777989317 58.974719121474422]  MomentsOfInertiaUnits=kg*mm^2  ProductsOfInertia=[-12.770089995694509 -9.4582724645364351 -6.681394862606262]  ProductsOfInertiaUnits=kg*mm^2  BasedOnType=Density  Density=1000  DensityUnits=kg/(m^3)  DoExposeReferenceFrame=on  SerializedFrames=<Frames/>  GraphicType=FromGeometry  MarkerShape=Sphere  MarkerSize=10  MarkerSizeUnits=m  GraphicVisPropType=SimpleVisualProperties  GraphicDiffuseColor=[0.792156862745098 0.81960784313725488 0.93333333333333335]  GraphicSpecularColor=[0.5 0.5 0.5 1.0]  GraphicAmbientColor=[0.15 0.15 0.15 1.0]  GraphicEmissiveColor=[0.0 0.0 0.0 1.0]  GraphicShininess=75  GraphicOpacity=1  GeometryShape=FromFile  RectangleSize=[1 1]  RectangleSizeUnits=m  BrickDimensions=[1 1 1]  BrickDimensionUnits=m  CylinderRadius=1  CylinderRadiusUnits=m  CylinderLength=1  CylinderLengthUnits=m  SphereRadius=1  SphereRadiusUnits=m  EllipsoidRadii=[1 1 1]  EllipsoidRadiiUnits=m  ExtrusionCrossSection=[1 1; -1 1; -1 -1; 1 -1]  ExtrusionCrossSectionUnits=m  ExtrusionLength=1  ExtrusionLengthUnits=m  PolygonNumSides=3  PolygonOuterRadius=1  PolygonOuterRadiusUnits=m  ExtGeomFileType=STL  ExtGeomFileName=\STL\carter transparent modif matlab_Défaut_sldprt.STL  ExtGeomFileUnits=mm  RevolutionCrossSection=[1 1; 1 -1; 2 -1; 2 1]  RevolutionCrossSectionUnits=m  RevolutionExtent=Full  RevolutionAngle=180  RevolutionAngleUnits=deg
  F : PMIOPort  Side=Left
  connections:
  Solid/RConn1 -- ReferenceFrame/RConn1 -- F/RConn1

== matlab function R19a_Asserv1_perturb_effort_boule/Calcul
consignes/AngleMoteur3 ==
function anglmot3  = fcn(x,y,z)
%#codegen
x = x/1000; y = y/1000; z = z/1000;
a = 0.06;
b = 0.1025;
c = 0.014;
d = 0.01125;
e = 0.01125;
f = 0.025 ;
r = 0.03723;
s = 0.02733;
phi1 = -0.252; %radians
pu1 = x*cos(phi1) + y*sin(phi1);
pv1 = -x*sin(phi1) + y*cos(phi1);
pw1 = z+0.082; 
theta11 = acos((s+pv1-f)/b);
equ10 = pu1-r+c;
equ11 = (pw1^2)+(equ10^2)+(a^2)+2*a*equ10-(d+e+b*sin(theta11))^2;
equ12 = (pw1^2)+(equ10^2)+(a^2)-2*a*equ10-(d+e+b*sin(theta11))^2;
equ13 = -4*a*pw1;
equ14 = (equ13^2)-4*equ11*equ12;
t1 = -(sqrt(equ14)+equ13)/(2*equ11);
anglmot3 = (atan(t1)*2+0.2073)*7.627;

== matlab function R19a_Asserv1_perturb_effort_boule/Calcul
consignes/AngleMoteur1 ==
function anglmot1  = fcn(x,y,z)
%#codegen
x = x/1000; y = y/1000; z = z/1000;
a = 0.06;
b = 0.1025;
c = 0.014;
d = 0.01125;
e = 0.01125;
f = 0.025 ;
r = 0.03723;
s = 0.02733;
phi1 = 1.842;
pu1 = x*cos(phi1) + y*sin(phi1);
pv1 = -x*sin(phi1) + y*cos(phi1);
pw1 = z+0.082;
theta11 = acos((s+pv1-f)/b);
equ10 = pu1-r+c;
equ11 = (pw1^2)+(equ10^2)+(a^2)+2*a*equ10-(d+e+b*sin(theta11))^2;
equ12 = (pw1^2)+(equ10^2)+(a^2)-2*a*equ10-(d+e+b*sin(theta11))^2;
equ13 = -4*a*pw1;
equ14 = (equ13^2)-4*equ11*equ12;
t1 = -(sqrt(equ14)+equ13)/(2*equ11);
anglmot1 = (atan(t1)*2+0.2073)*7.627; %7.627

== matlab function R19a_Asserv1_perturb_effort_boule/Calcul
consignes/AngleMoteur2 ==
function anglmot2 = fcn(x,y,z)
%#codegen
x = x/1000; y = y/1000; z = z/1000;
a = 0.06;
b = 0.1025;
c = 0.014;
d = 0.01125;
e = 0.01125;
f = 0.025 ;
r = 0.03723;
s = 0.02733;
phi1 = 3.937; %radians
pu1 = x*cos(phi1) + y*sin(phi1);
pv1 = -x*sin(phi1) + y*cos(phi1);
pw1 = z+0.082; 
theta11 = acos((s+pv1-f)/b);
equ10 = pu1-r+c;
equ11 = (pw1^2)+(equ10^2)+(a^2)+2*a*equ10-(d+e+b*sin(theta11))^2;
equ12 = (pw1^2)+(equ10^2)+(a^2)-2*a*equ10-(d+e+b*sin(theta11))^2;
equ13 = -4*a*pw1;
equ14 = (equ13^2)-4*equ11*equ12;
t1 = -(sqrt(equ14)+equ13)/(2*equ11);
anglmot2 = (atan(t1)*2+0.2073)*7.627;
